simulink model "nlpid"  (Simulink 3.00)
settings: Solver=ode45  StartTime=0.0  StopTime=300  RelTol=1e-6  AbsTol=1e-6
libraries: simulink_extras x1

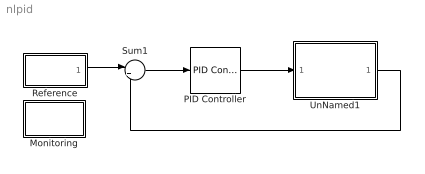
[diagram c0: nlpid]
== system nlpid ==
  Monitoring : Subsystem
  PID Controller : simulink_extras/Additional Linear/PID Controller  P=0.03  I=0  D=0
  Reference : Subsystem
  Sum1 : Sum  Inputs=|+-  SaturateOnIntegerOverflow=on
  UnNamed1 : Subsystem
      mask help: Non-linear 3-rd order process
      mask init:
      | ic = @1;
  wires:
  Sum1/1 -> PID Controller/1
  Reference/1(Out1) -> Sum1/1
  PID Controller/1 -> UnNamed1/1(in_1)
  UnNamed1/1(out_1) -> Sum1/2

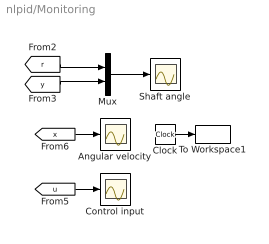
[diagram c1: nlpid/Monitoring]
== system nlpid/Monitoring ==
  Angular velocity : Scope
  Clock : Clock
  Control input : Scope
  Mux : Mux  Inputs=2
  Shaft angle : Scope
  To Workspace1 : ToWorkspace  VariableName=t  SampleTime=0.1  SaveFormat=Matrix
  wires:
  [y] -> Mux/2
  [r] -> Mux/1
  Mux/1 -> Shaft angle/1
  [u] -> Control input/1
  Clock/1 -> To Workspace1/1
  [x] -> Angular velocity/1

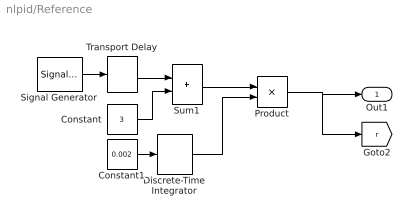
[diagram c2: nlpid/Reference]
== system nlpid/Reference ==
  Constant : Constant  Value=3
  Constant1 : Constant  Value=0.002
  Discrete-Time Integrator : DiscreteIntegrator  IntegratorMethod=ForwardEuler  ExternalReset=none  InitialConditionSource=internal  InitialCondition=1  LimitOutput=off  UpperSaturationLimit=inf  LowerSaturationLimit=-inf  ShowSaturationPort=off  ShowStatePort=off  SampleTime=[50 10]
  Product : Product  Inputs=2  SaturateOnIntegerOverflow=on
  Signal Generator : SignalGenerator  WaveForm=square  Amplitude=1  Frequency=1/100  Units=Hertz
  Sum1 : Sum  Inputs=++  SaturateOnIntegerOverflow=on
  Transport Delay : TransportDelay  DelayTime=10  InitialInput=0  BufferSize=1024
  Out1 : Outport  Port=1
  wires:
  Signal Generator/1 -> Transport Delay/1
  Transport Delay/1 -> Sum1/1
  Constant/1 -> Sum1/2
  Sum1/1 -> Product/1
  Product/1 -> Out1/1, [r]
  Constant1/1 -> Discrete-Time Integrator/1
  Discrete-Time Integrator/1 -> Product/2

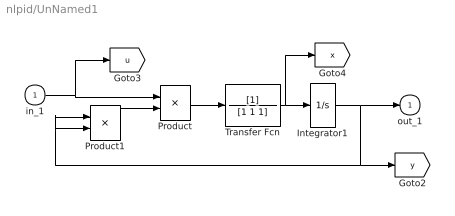
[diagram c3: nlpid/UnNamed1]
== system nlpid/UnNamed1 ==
  in_1 : Inport  Port=1  PortWidth=-1  SampleTime=-1  DataType=auto
  Integrator1 : Integrator  ExternalReset=none  InitialConditionSource=internal  InitialCondition=ic  LimitOutput=off  UpperSaturationLimit=inf  LowerSaturationLimit=-inf  ShowSaturationPort=off  ShowStatePort=off  AbsoluteTolerance=auto
  Product : Product  Inputs=2  SaturateOnIntegerOverflow=on
  Product1 : Product  Inputs=2  SaturateOnIntegerOverflow=on
  Transfer Fcn : TransferFcn  Numerator=[1]  Denominator=[1 1 1]
  out_1 : Outport  Port=1
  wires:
  Product/1 -> Transfer Fcn/1
  Product1/1 -> Product/2
  Integrator1/1 -> out_1/1, Product1/1, Product1/2, [y]
  Transfer Fcn/1 -> Integrator1/1, [x]
  in_1/1 -> Product/1, [u]
